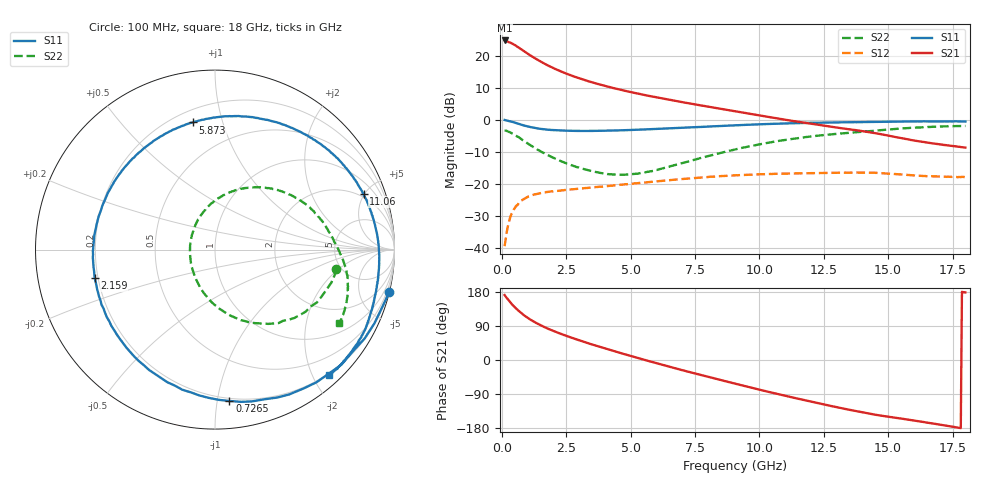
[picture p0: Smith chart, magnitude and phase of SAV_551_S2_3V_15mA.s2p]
! Data provided by Modelithics, Inc.  Tampa, Florida USA, June 2008
!Model SAV-551+
!VAR V_out= 3
!VAR I_out= 15
!VAR V_in= 0.3190
!VAR I_in= 0.8429
!BEGIN ACDATA
# GHZ S MA R 50
! Scattering Parameters
!% F n11x n11y n21x n21y n12x n12y n22x n22y
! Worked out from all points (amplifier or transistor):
!   401 points, 100 MHz to 18 GHz, reference 50 ohm
!   highest |S21| = 24.8 dB at 100 MHz (marker M1)
!   |S21| within 3 dB of that: start of sweep to 789.5 MHz
!   unconditionally stable (mu >= 1): 4.507 GHz to 10.33 GHz; 10.38278 GHz to 10.3975 GHz
!   at 3.054 GHz: K = 0.79, MSG = 17.1 dB, |S12| = -21.4 dB
!   at 9.05 GHz: K = 1.06, MAG = 8.5 dB, |S12| = -17.3 dB
!   at 18 GHz: K = 0.86, MSG = 4.6 dB, |S12| = -17.8 dB
!   lowest NFmin = 0.07 dB at 500 MHz
!   S11 on the Smith chart (normalised r, x): 100 MHz: 0.02, -8.37; 726.5 MHz: 0.18, -1.08; 2.159 GHz: 0.19, -0.11; 5.873 GHz: 0.27, +0.80; 11.06 GHz: 1.74, +4.93; 18 GHz: 0.17, -2.26
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0.1  0.9993 -13.6  17.4 171.4  0.01071 83.4  0.6829 -9.2
0.14475  0.9855 -18.9  16.85 167.0  0.014 78.5  0.6809 -12.3
0.23425  0.9696 -30.8  16.61 159.5  0.02257 72.6  0.6586 -20.1
0.32375  0.9526 -42.3  16.12 152.2  0.03099 66.0  0.6395 -27.4
0.41325  0.9305 -52.7  15.42 145.1  0.03603 62.2  0.6114 -34.5
0.5475  0.8944 -67.1  14.32 135.9  0.04574 54.9  0.5675 -43.5
0.7265  0.8469 -84.6  12.82 125.0  0.05445 46.4  0.5093 -54.4
0.995  0.7904 -106.4  10.84 111.3  0.06282 36.8  0.4298 -67.6
1.30825  0.747 -126.8  9.031 98.5  0.06924 29.2  0.3579 -80.3
1.711  0.7107 -147.9  7.339 84.9  0.07486 21.7  0.2918 -94.0
2.1585  0.6887 -166.7  6.026 72.3  0.07811 15.9  0.2395 -107.3
2.606  0.6779 177.7  5.085 61.1  0.08175 11.6  0.2026 -119.7
3.09825  0.6731 162.8  4.327 49.8  0.08533 7.4  0.1747 -133.6
4.396  0.6851 130.3  3.094 22.5  0.09551 -2.1  0.1401 -174.6
5.87275  0.7192 99.8  2.304 -6.1  0.1088 -13.2  0.1606 138.2
6.0965  0.7269 95.7  2.214 -10.2  0.1109 -15.0  0.1695 132.2
7.439  0.7684 72.7  1.763 -34.5  0.1236 -27.0  0.2368 100.8
9.05  0.8223 48.3  1.364 -62.3  0.1364 -42.7  0.3454 71.8
11.06375  0.8835 20.5  0.9993 -95.3  0.1456 -64.8  0.4911 41.4
12.04825  0.9021 8.3  0.8645 -110.4  0.148 -75.7  0.5549 28.7
15.0465  0.9378 -22.9  0.5651 -150.1  0.145 -106.3  0.7105 -3.9
18  0.9444 -47.6  0.3699 178.3  0.1282 -131.3  0.8055 -30.7
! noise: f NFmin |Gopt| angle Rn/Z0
0.5  0.073  0.3822  23.41  0.074
0.7  0.104  0.3903  33.53  0.068
0.9  0.135  0.3983  43.52  0.061
1  0.151  0.4022  48.46  0.059
1.9  0.291  0.4367  91.46  0.041
2.4  0.368  0.455  114.2  0.038
3  0.462  0.4761  140.3  0.039
3.9  0.602  0.5061  177.3  0.053
5  0.773  0.54  -141.2  0.09
6  0.928  0.5681  -106.9  0.141
